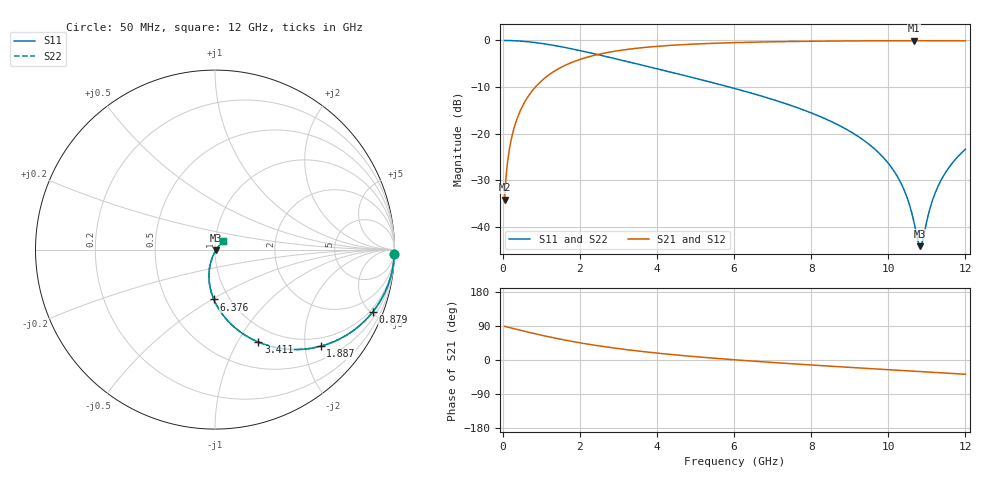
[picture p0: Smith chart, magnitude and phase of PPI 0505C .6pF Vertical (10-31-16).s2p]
# GHz S MA R 50
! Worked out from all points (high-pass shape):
!   1601 points, 50 MHz to 12 GHz, reference 50 ohm
!   highest |S21| = -0.06 dB at 10.66 GHz (marker M1); lowest = -34.2 dB at 50 MHz (marker M2)
!   |S21| within 3 dB of the highest: 2.443 GHz to end of sweep
!   lowest |S11| = -44.1 dB at 10.83 GHz (marker M3), VSWR 1.01, Z = 50.5 - j0.337 ohm
!   |S11| at or under -10 dB: 5.881 GHz to end of sweep
!   |S22| runs from -44.1 to 0.0 dB; largest |S21 - S12| = 0
!   S11 on the Smith chart (normalised r, x): 50 MHz: 1, -90; 879 MHz: 0.79, -5.12; 1.887 GHz: 0.79, -2.34; 3.411 GHz: 0.80, -1.23; 6.376 GHz: 0.85, -0.51; 12 GHz: 1.09, +0.11
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0.05  0.9998 -1.3  0.01957 88.7  0.01957 88.7  0.9998 -1.3
0.1769688  0.9976 -4.5  0.06911 85.5  0.06911 85.5  0.9976 -4.5
0.318875  0.9922 -8.0  0.1239 81.9  0.1239 81.9  0.9922 -8.0
0.5504062  0.9774 -13.8  0.2109 76.2  0.2109 76.2  0.9774 -13.8
0.8790313  0.9449 -21.6  0.3266 68.3  0.3266 68.3  0.9449 -21.6
1.887312  0.7973 -42.5  0.6018 47.4  0.6018 47.4  0.7973 -42.5
2.044156  0.7721 -45.2  0.6336 44.6  0.6336 44.6  0.7721 -45.2
3.410938  0.5697 -64.8  0.8189 24.9  0.8189 24.9  0.5697 -64.8
4.038312  0.4927 -71.8  0.8669 17.9  0.8669 17.9  0.4927 -71.8
6.025  0.3048 -88.8  0.948 0.5  0.948 0.5  0.3048 -88.8
6.376031  0.2778 -91.3  0.9561 -2.1  0.9561 -2.1  0.2778 -91.3
8.019156  0.1661 -101.6  0.9807 -13.3  0.9807 -13.3  0.1661 -101.6
9.221625  0.09332 -107.5  0.9896 -20.8  0.9896 -20.8  0.09332 -107.5
10.01331  0.04744 -108.6  0.9924 -25.7  0.9924 -25.7  0.04744 -108.6
10.39422  0.02584 -104.5  0.993 -27.9  0.993 -27.9  0.02584 -104.5
10.65563  0.01181 -88.3  0.9931 -29.5  0.9931 -29.5  0.01181 -88.3
10.82741  0.00622 -32.5  0.9931 -30.5  0.9931 -30.5  0.00622 -32.5
10.89462  0.007245 -0.6  0.9931 -31.0  0.9931 -31.0  0.007245 -0.6
11.12616  0.01816 37.1  0.9928 -32.3  0.9928 -32.3  0.01816 37.1
11.31288  0.02854 43.4  0.9924 -33.5  0.9924 -33.5  0.02854 43.4
11.61909  0.04603 46.4  0.9916 -35.3  0.9916 -35.3  0.04603 46.4
12  0.06813 46.6  0.9901 -37.6  0.9901 -37.6  0.06813 46.6
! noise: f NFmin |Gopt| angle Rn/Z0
0.05  0.001624  0.9807  1.137  0.01924
1.372  0.005859  0.7779  7.524  0.005378
2.701  0.009111  0.7189  10.73  0.006358
4.031  0.01201  0.6853  14.02  0.0073
5.36  0.01475  0.6632  17.32  0.008206
6.682  0.01742  0.6482  20.6  0.00911
8.012  0.02011  0.6381  23.85  0.01006
9.341  0.02287  0.6321  27.05  0.01107
10.67  0.02573  0.6295  30.2  0.01219
12  0.02876  0.63  33.28  0.01345
